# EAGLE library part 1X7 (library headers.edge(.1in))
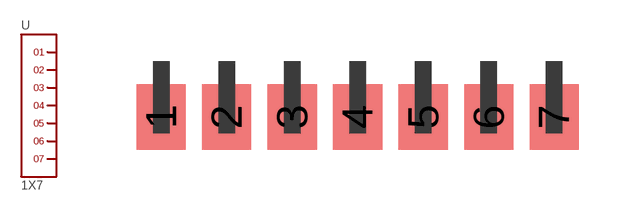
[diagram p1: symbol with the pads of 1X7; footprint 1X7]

Designator prefix -

## 1X7  [1X7]
1  1
2  2
3  3
4  4
5  5
6  6
7  7

## Footprint 1X7 (pad centres in mm)
smd 1.905 x 2.54: 1 0,-2.159; 2 2.54,-2.159; 3 5.08,-2.159; 4 7.62,-2.159; 5 10.16,-2.159; 6 12.7,-2.159; 7 15.24,-2.159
